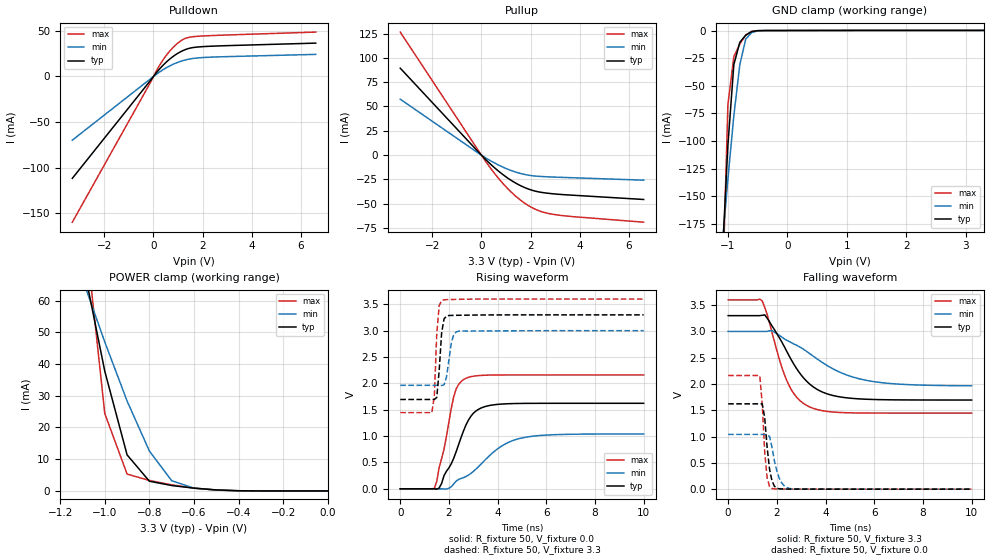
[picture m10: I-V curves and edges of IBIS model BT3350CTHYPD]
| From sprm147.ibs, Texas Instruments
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[Model]   BT3350CTHYPD
Model_type   I/O
Vinh = 2.00
Vinl = 0.80
Enable   Active-Low
Polarity   Non-Inverting
| signals   A, GZ, Y
Vmeas = 1.5
|   typ   min   max
C_comp   1.3064919p   1.2567267p   1.3809238p
|   typ   min   max
[Temperature Range]   25   -40   125
|   typ   min   max
[Voltage Range]   3.30V   3.00V   3.60V
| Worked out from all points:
|   slope of the pulldown table from 0 to 0.495 V, typ, clamps not added: 32.7 ohm
|   slope of the pullup table from 0 to 0.495 V, typ, clamps not added: 40.8 ohm
|   GND clamp passes 1 mA (typ) near -0.60 V on its own axis
|   POWER clamp passes 1 mA (typ) near -0.62 V on its own axis
|   rising waveform, R_fixture 50, V_fixture 0.0: 20-80 % time 909ps typ, 1.67ns min, 575ps max; typ from 0 V to 1.62 V
|   falling waveform, R_fixture 50, V_fixture 3.3: 20-80 % time 1.34ns typ, 2.29ns min, 922ps max; typ from 3.3 V to 1.7 V
|   rising waveform, R_fixture 50, V_fixture 3.3: 20-80 % time 152ps typ, 198ps min, 133ps max; typ from 1.7 V to 3.3 V
|   falling waveform, R_fixture 50, V_fixture 0.0: 20-80 % time 213ps typ, 315ps min, 177ps max; typ from 1.62 V to 0 V
[Pulldown]
|   Voltage   I(typ)   I(min)   I(max)
-3.3V     -111.9mA   -69.94mA   -160.1mA
-200mV    -7.006mA   -4.258mA   -10.31mA
200mV     6.74mA     4.038mA    10.03mA
400mV     12.65mA    7.621mA    18.63mA
600mV     17.74mA    10.75mA    25.92mA
1V        25.63mA    15.66mA    36.92mA
1.3V      29.62mA    18.2mA     41.96mA
1.7V      32.11mA    20.12mA    43.97mA
2.7V      33.64mA    21.61mA    45.32mA
6.6V      36.68mA    24.3mA     48.79mA
[GND_clamp]
|   Voltage   I(typ)   I(min)   I(max)
-3.3V     -3.112A    -1.738A    -6.702A
-1.1V     -211.3mA   -197.1mA   -254.9mA
-1V       -103.9mA   -134.6mA   -67.28mA
-900mV    -30.88mA   -77.09mA   -23.7mA
-800mV    -10.69mA   -31.04mA   -12.21mA
-700mV    -4.206mA   -7.793mA   -4.159mA
-600mV    -961uA     -1.874mA   -663.9uA
-500mV    -137.2uA   -368.7uA   -104.9uA
-400mV    -40.82uA   -64.04uA   -57.02uA
3.3V      101.5uA    59.92uA    182uA
[Pullup]
|   Voltage   I(typ)   I(min)   I(max)
-3.3V     89.43mA    57.53mA    126.5mA
300mV     -7.587mA   -4.746mA   -10.95mA
700mV     -16.56mA   -10.26mA   -24mA
1V        -22.37mA   -13.74mA   -32.59mA
1.6V      -31.53mA   -18.93mA   -46.5mA
1.9V      -34.78mA   -20.58mA   -51.75mA
2.2V      -37.11mA   -21.57mA   -55.79mA
2.5V      -38.57mA   -22.09mA   -58.61mA
2.9V      -39.77mA   -22.57mA   -60.85mA
3.7V      -41.24mA   -23.28mA   -63.23mA
6.6V      -45.65mA   -25.8mA    -69.01mA
[POWER_clamp]
|   Voltage   I(typ)   I(min)   I(max)
-3.3V     981.8mA    550.5mA    2.111A
-1.1V     72.59mA    66.83mA    89.79mA
-1V       37.73mA    46.94mA    24.4mA
-900mV    11.36mA    28.34mA    5.309mA
-800mV    3.058mA    12.55mA    3.288mA
-700mV    1.696mA    3.224mA    1.922mA
-600mV    874.7uA    863.1uA    893.4uA
-500mV    320.1uA    290.1uA    245.7uA
-400mV    56.01uA    61.69uA    23.4uA
0V        1pA        1pA        1pA
[Ramp]
|   I(typ)   I(min)   I(max)
dV/dt_r   0.974/0.908n   0.625/1.663n   1.296/0.575n
dV/dt_f   0.963/1.331n   0.620/2.293n   1.292/0.920n
[Rising Waveform]
R_fixture = 50
V_fixture = 0.0
|  pu_on
|  TIME   V(typ)   V(min)   V(max)
0s        18nV       187nV      1nV
1.4ns     480.2uV    -5.966uV   7.555mV
1.6ns     16.27mV    65.41uV    410.1mV
1.8ns     252.3mV    -2.809mV   757.3mV
2.2ns     584.2mV    94.34mV    1.753V
2.4ns     842.2mV    178mV      1.983V
2.7ns     1.212V     232.7mV    2.098V
3.3ns     1.529V     461.1mV    2.151V
4.9ns     1.62V      954.7mV    2.161V
10ns      1.623V     1.041V     2.161V
[Falling Waveform]
R_fixture = 50
V_fixture = 3.3
V_fixture_min = 3.0
V_fixture_max = 3.6
|  pd_on
|  TIME   V(typ)   V(min)   V(max)
0s        3.3V       3V         3.6V
1.4ns     3.307V     3V         3.579V
1.6ns     3.255V     3V         3.327V
2.1ns     2.882V     2.928V     2.474V
2.4ns     2.628V     2.833V     2.075V
2.8ns     2.301V     2.739V     1.756V
3.3ns     2.019V     2.595V     1.575V
4.2ns     1.794V     2.315V     1.471V
5.7ns     1.71V      2.067V     1.448V
10ns      1.695V     1.967V     1.446V
[Rising Waveform]
R_fixture = 50
V_fixture = 3.3
V_fixture_min = 3.0
V_fixture_max = 3.6
|  pd_off
|  TIME   V(typ)   V(min)   V(max)
0s        1.695V     1.963V     1.446V
1.3ns     1.695V     1.963V     1.444V
1.4ns     1.695V     1.963V     1.764V
1.5ns     1.733V     1.963V     2.936V
1.6ns     2.244V     1.964V     3.477V
1.7ns     2.959V     1.961V     3.57V
1.9ns     3.278V     2.12V      3.589V
2.2ns     3.291V     2.931V     3.593V
2.4ns     3.293V     2.99V      3.595V
10ns      3.3V       3V         3.6V
[Falling Waveform]
R_fixture = 50
V_fixture = 0.0
|  pu_off
|  TIME   V(typ)   V(min)   V(max)
0s        1.623V     1.041V     2.161V
1.3ns     1.622V     1.041V     2.158V
1.4ns     1.621V     1.041V     1.62V
1.5ns     1.368V     1.041V     716.9mV
1.6ns     801.6mV    1.042V     219.4mV
1.7ns     379.3mV    1.002V     47.99mV
1.8ns     159.4mV    799.5mV    12.31mV
2.1ns     7.067mV    205.6mV    2.367mV
2.5ns     2.212mV    15.36mV    1.227mV
10ns      354nV      14.56uV    692nV
